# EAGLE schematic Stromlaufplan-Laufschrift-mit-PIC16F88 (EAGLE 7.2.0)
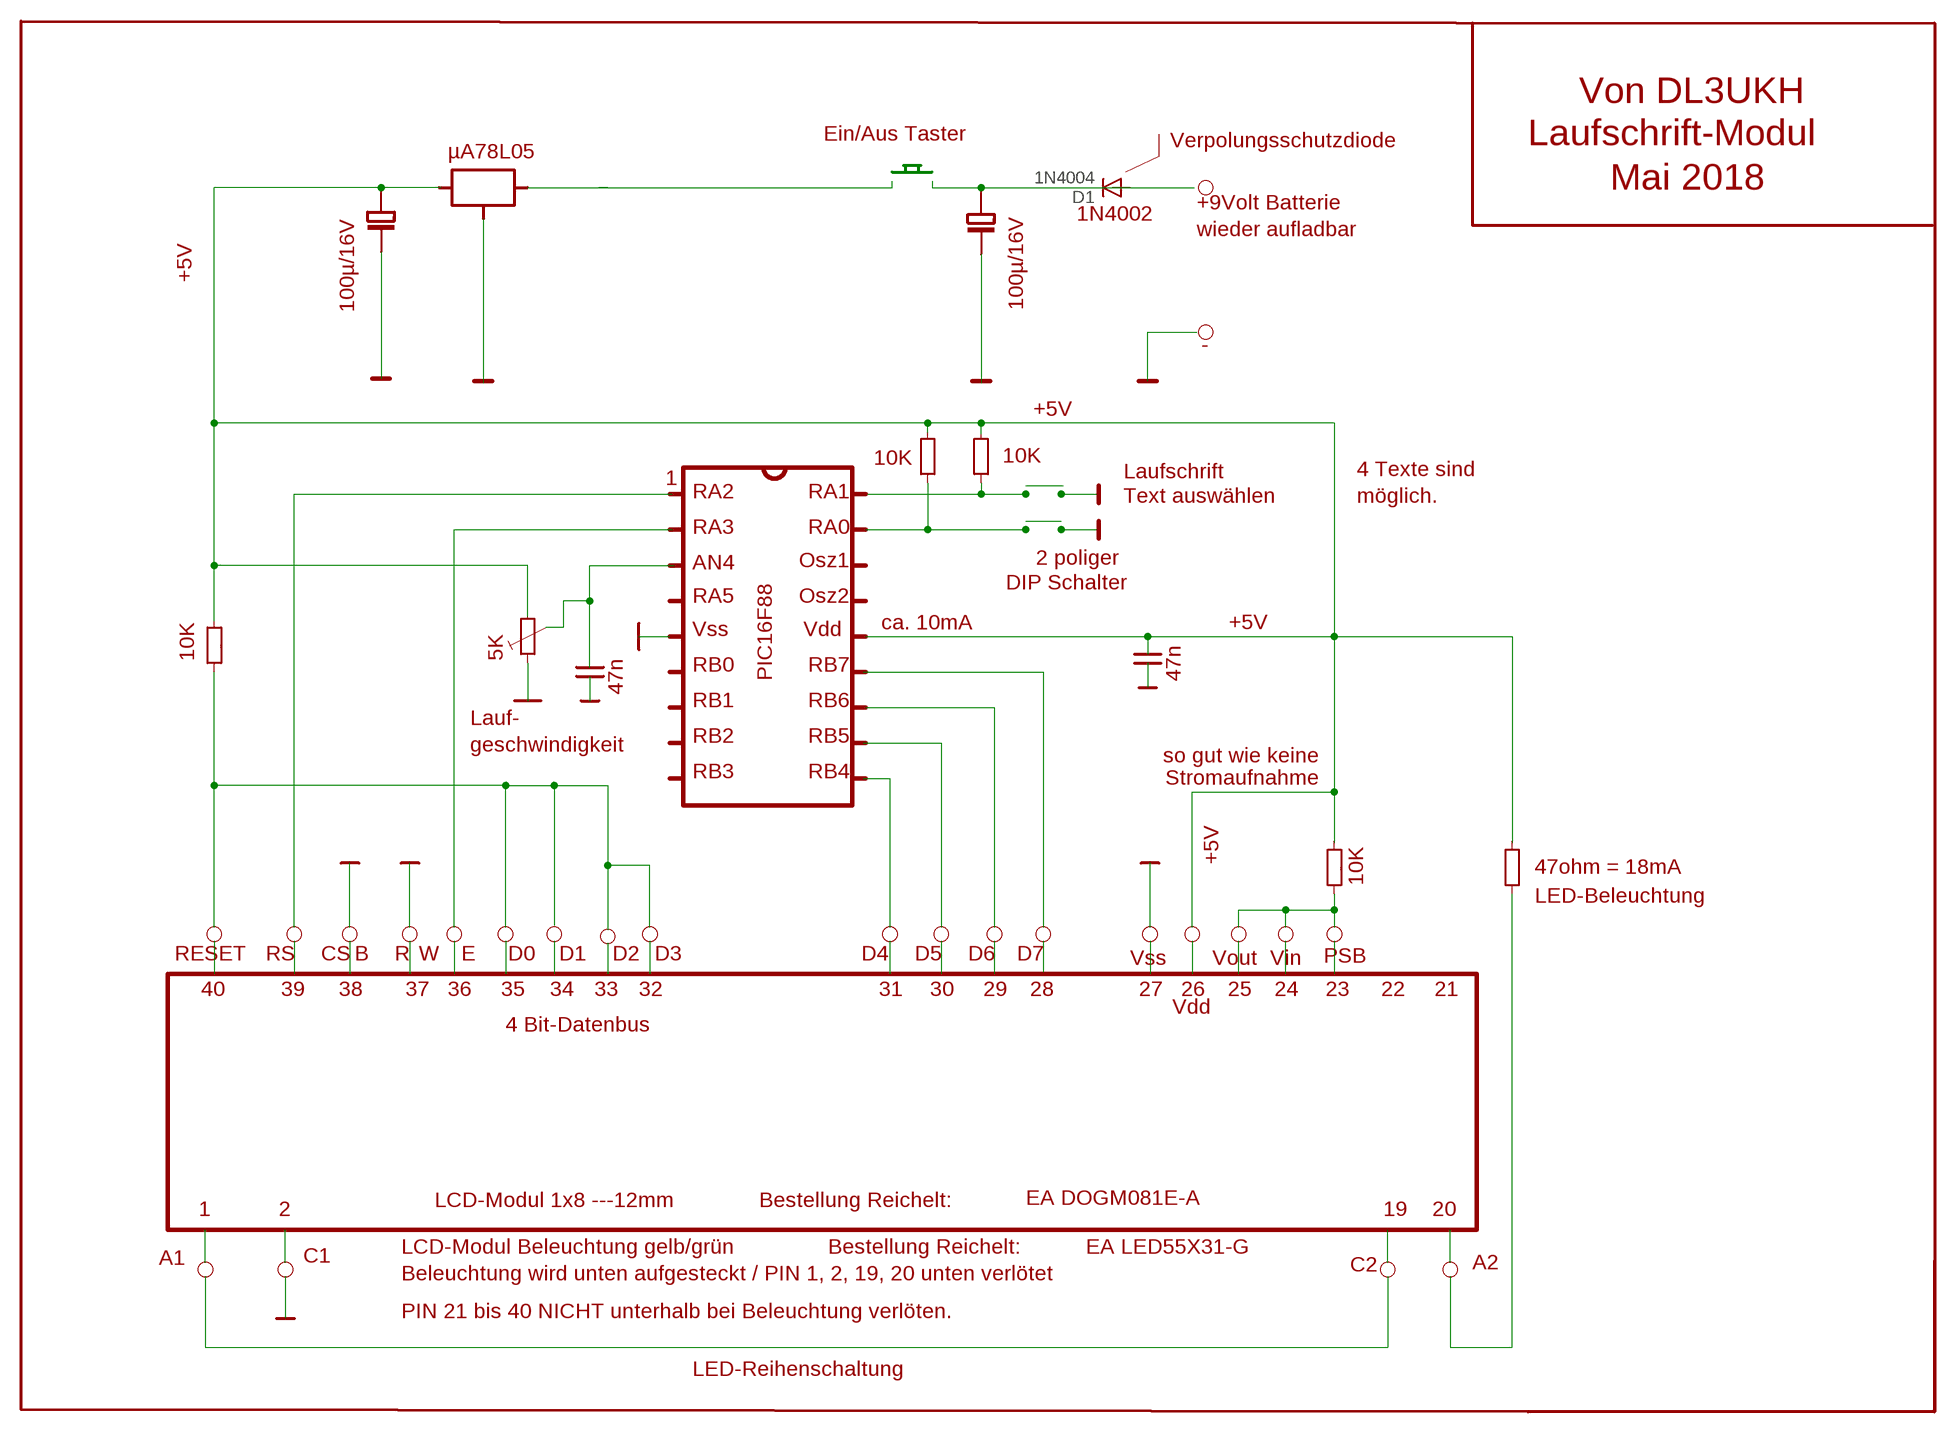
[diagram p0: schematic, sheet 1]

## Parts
D1  1N4004  [DO41-10]

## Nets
N$48: D1.A D1.C

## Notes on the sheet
- Von DL3UKH
- Ein/Aus Taster | Laufschrift-Modul
- Verpolungsschutzdiode
- µA78L05
- Mai 2018
- +9Volt Batterie
- 1N4002
- wieder aufladbar
- +5V
- 100µ/16V | 100µ/16V
- -
- +5V
- 10K | 10K
- Laufschrift | 4 Texte sind
- 1
- RA2 | RA1 | Text auswählen | möglich.
- RA3 | RA0
- 2 poliger
- AN4 | Osz1
- DIP Schalter
- RA5 | Osz2
- +5V
- 5K | ca. 10mA
- Vss | Vdd
- 47n
- 10K | 47n
- RB0 | RB7
- PIC16F88
- RB1 | RB6
- Lauf-
- RB2 | RB5 | so gut wie keine
- geschwindigkeit
- Stromaufnahme
- RB3 | RB4
- +5V
- 47ohm = 18mA
- 10K
- LED-Beleuchtung
- RESET | RS | CS | B | R | W | E | D0 | D1 | D2 | D3 | D4 | D5 | D6 | D7 | Vss | Vout | Vin | PSB
- 40 | 39 | 38 | 37 | 36 | 35 | 34 | 33 | 32 | 31 | 30 | 29 | 28 | 27 | 26 | 25 | 24 | 23 | 22 | 21
- Vdd
- 4 Bit-Datenbus
- LCD-Modul 1x8 ---12mm | Bestellung Reichelt: | EA DOGM081E-A
- 1 | 2 | 19 | 20
- LCD-Modul Beleuchtung gelb/grün | Bestellung Reichelt: | EA LED55X31-G
- A1 | C1
- C2 | A2
- Beleuchtung wird unten aufgesteckt / PIN 1, 2, 19, 20 unten verlötet
- PIN 21 bis 40 NICHT unterhalb bei Beleuchtung verlöten.
- LED-Reihenschaltung

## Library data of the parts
D1 = diode:1N4004: DIODE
